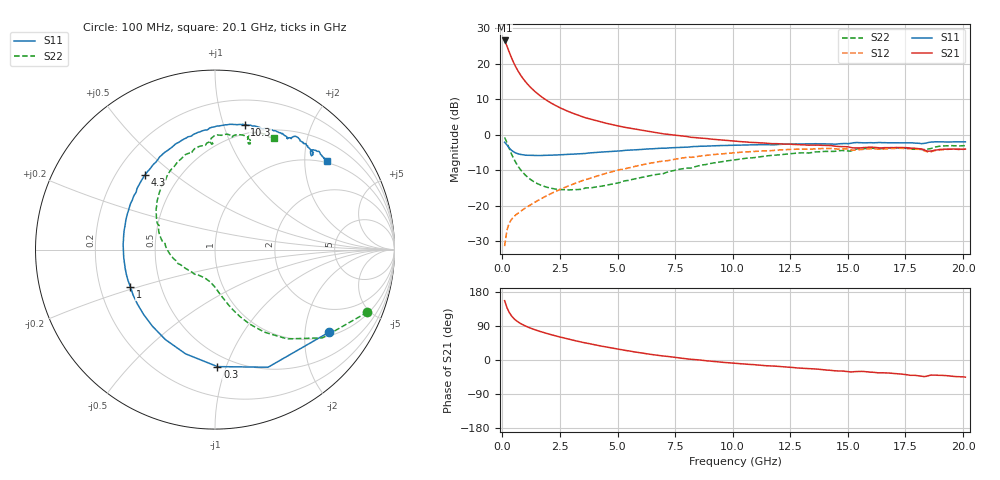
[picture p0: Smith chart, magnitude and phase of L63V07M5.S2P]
!  Infineon Technologies AG
! BFR380L3 , PF131585-7, No.6, Th 09.10.01, soldered on pcb-board, measured with PP GSG850
!  Vce=3.0 V,  Ic=7.5 mA
! Common Emitter S-Parameters:  15. November 2001
#  GHz  S  MA  R  50
! f  S11  S21  S12  S22
! GHz  Mag  Ang  Mag  Ang  Mag  Ang  Mag  Ang
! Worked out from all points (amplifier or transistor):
!   201 points, 100 MHz to 20.1 GHz, reference 50 ohm
!   highest |S21| = 26.6 dB at 100 MHz (marker M1)
!   |S21| within 3 dB of that: start of sweep to 284.3 MHz
!   unconditionally stable (mu >= 1): 2.029 GHz to 4.498 GHz
!   at 3.4 GHz: K = 1.03, MAG = 8.1 dB, |S12| = -13.1 dB
!   at 10.1 GHz: K = 0.94, MSG = 1.6 dB, |S12| = -5.1 dB
!   at 20.1 GHz: K = 0.99, MSG = 0.0 dB, |S12| = -4.1 dB
!   S11 on the Smith chart (normalised r, x): 100 MHz: 1.12, -2.68; 300 MHz: 0.41, -0.93; 1 GHz: 0.33, -0.19; 4.3 GHz: 0.32, +0.39; 10.3 GHz: 0.41, +1.18; 20.1 GHz: 0.96, +2.57
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0.1  0.785 -35.8  21.31 156.6  0.02695 73.1  0.9181 -22.3
0.2  0.7189 -65.7  17.82 138.4  0.04523 60.1  0.7749 -39.4
0.3  0.6521 -88.8  14.63 125.6  0.05695 52.8  0.6393 -51.1
0.4  0.6036 -105.7  12.14 116.3  0.06423 48.8  0.5344 -59.2
0.5  0.5723 -119.0  10.25 109.5  0.07008 46.9  0.4565 -65.1
0.6  0.5509 -129.4  8.836 104.1  0.07502 46.4  0.3984 -69.5
0.7  0.5372 -137.9  7.746 99.7  0.07933 46.4  0.3538 -73.1
0.8  0.5281 -144.9  6.879 95.9  0.08385 46.9  0.3193 -76.1
1  0.5152 -156.1  5.619 89.8  0.09274 48.3  0.2705 -80.9
1.2  0.5128 -164.8  4.745 84.7  0.1017 49.6  0.2377 -85.1
1.4  0.51 -171.7  4.111 80.2  0.1114 51.1  0.2152 -88.9
1.9  0.5127 174.3  3.095 70.6  0.137 53.2  0.1836 -97.9
2.6  0.525 159.6  2.322 59.2  0.175 53.9  0.1688 -111.0
3.5  0.5428 144.4  1.784 46.4  0.2273 52.4  0.1722 -127.2
4.3  0.5706 133.2  1.509 36.7  0.2737 49.6  0.1887 -143.8
5.3  0.6019 120.8  1.276 25.6  0.3306 44.4  0.2239 -161.1
6.8  0.6422 104.4  1.057 11.9  0.418 35.2  0.2789 174.2
10.1  0.7117 78.2  0.8113 -8.7  0.5585 13.4  0.4448 134.1
10.3  0.7145 76.7  0.8026 -9.6  0.5653 12.1  0.453 131.9
13.5  0.7448 60.1  0.7151 -23.4  0.632 -8.5  0.5662 102.4
16.8  0.7707 47.7  0.6578 -34.5  0.6359 -25.0  0.6512 79.2
20.1  0.7945 38.2  0.6283 -45.2  0.6263 -39.0  0.7025 62.2
